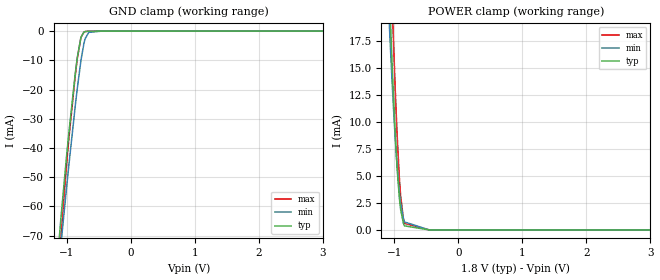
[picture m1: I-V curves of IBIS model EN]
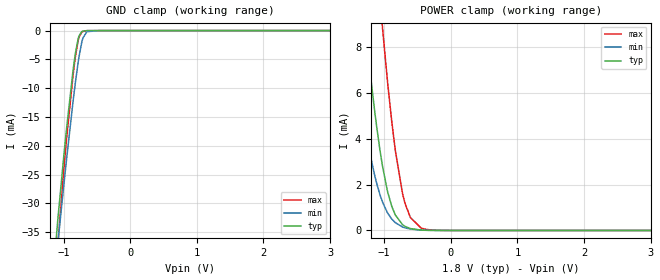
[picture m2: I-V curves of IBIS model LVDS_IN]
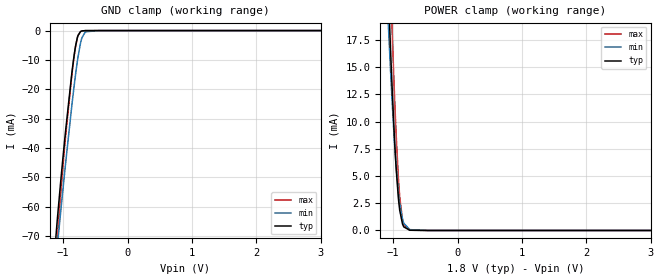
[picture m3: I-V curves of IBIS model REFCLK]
|Texas Instruments Incorporated
| High Performance Single-Synchronous Step-Down Controller
| with Differential Voltage Feedback
| Marketing part#   Digital Voltage Range   Package-type   #pins
| SN65DSI85ZQER   1.65V-1.95   PBGA   64
| SN65DSI85ZQET   1.65V-1.95   PBGA   64
[IBIS Ver]   4.1
[File name]   sn65dsi84.ibs
[File Rev]   1.0
[Date]   1/28/2013
[Source]
| Texas Instruments Incorporated.
| Analog-eLab Design Center, HPA
| 12500 TI Blvd
| Dallas, TX -75243
| e-mail: elab_scm_ibis@list.ti.com
[Notes]   Revision History:
| Rev 1.0: 1/28/2013
| - Initial version of the model
| - Model generated from simulations in TISPICE
| - C_comp although listed in numerical order of value are
|   obtained from varying PVT conditions. For PVT conditions for
|   each specific value refer the buffer description under
|   respective [Model]. IBIS model user is responsible for using
|   appropriate C_comp to simulate for Signal Integrity.
| - Warnings regarding combined Non-monotonicity of various models have been
|   reviewd and considered minor and can be ignored.
| - LVDS outputs have sub models depending on the drive strength/on-chip termination
|   and common mode output level.
|   Please refer to the [Model Selector] section for details.
[Disclaimer]
| This model is designed as an aid for customers of Texas Instruments.
| TI and its licensors and suppliers make no warranties, either expressed
| or implied, with respect to this  model, including the warranties of
| merchantability or fitness for a particular purpose. The model is
| provided solely on an "as is" basis. The entire risk as to its quality
| and performance is with the customer.
[Copyright]
 (C) Copyright 2013 Texas Instruments Incorporated.All rights reserved.
|   SN65DSI84
[Component]   SN65DSI84
[Manufacturer]   TI
[Package]
| variable   typ   min   max
R_pkg   0.1   0.08   0.12
L_pkg   0.7nH   0.56nH   0.84nH
C_pkg   0.1pF   0.08pF   0.12pF
[Pin]  signal_name   model_name   R_pin   L_pin   C_pin
A1   ADDR   ADDR   NA   NA   NA
A2   GND   GND   NA   NA   NA
A3   B_Y0N   LVDS_DATA   NA   NA   NA
A4   B_Y1N   LVDS_DATA   NA   NA   NA
A5   B_Y2N   LVDS_DATA   NA   NA   NA
A6   B_CLKN   LVDS_CLK   NA   NA   NA
A7   B_Y3N   LVDS_DATA   NA   NA   NA
A8   GND   GND   NA   NA   NA
A9   VCC   POWER   NA   NA   NA
B1   EN   EN   NA   NA   NA
B2   RSVD2   NC   NA   NA   NA
B3   B_Y0P   LVDS_DATA   NA   NA   NA
B4   B_Y1P   LVDS_DATA   NA   NA   NA
B5   B_Y2P   LVDS_DATA   NA   NA   NA
B6   B_CLKP   LVDS_CLK   NA   NA   NA
B7   B_Y3P   LVDS_DATA   NA   NA   NA
B8   VCC   POWER   NA   NA   NA
B9   GND   GND   NA   NA   NA
C1   NC   NC   NA   NA   NA
C2   NC   NC   NA   NA   NA
C8   A_Y0P   LVDS_DATA   NA   NA   NA
C9   A_Y0N   LVDS_DATA   NA   NA   NA
D1   NC   NC   NA   NA   NA
D2   NC   NC   NA   NA   NA
D5   GND   GND   NA   NA   NA
D6   VCC   POWER   NA   NA   NA
D8   A_Y1P   LVDS_DATA   NA   NA   NA
D9   A_Y1N   LVDS_DATA   NA   NA   NA
E1   NC   NC   NA   NA   NA
E2   NC   NC   NA   NA   NA
E4   GND   GND   NA   NA   NA
E5   VCC   POWER   NA   NA   NA
E6   VCC   POWER   NA   NA   NA
E8   A_Y2P   LVDS_DATA   NA   NA   NA
E9   A_Y2N   LVDS_DATA   NA   NA   NA
F1   NC   NC   NA   NA   NA
F2   NC   NC   NA   NA   NA
F4   GND   GND   NA   NA   NA
F5   GND   GND   NA   NA   NA
F6   VCC   POWER   NA   NA   NA
F8   A_CLKP   LVDS_CLK   NA   NA   NA
F9   A_CLKN   LVDS_CLK   NA   NA   NA
G1   NC   NC   NA   NA   NA
G2   NC   NC   NA   NA   NA
G8   A_Y3P   LVDS_DATA   NA   NA   NA
G9   A_Y3N   LVDS_DATA   NA   NA   NA
H1   SCL   SCL   NA   NA   NA
H2   REFCLK   REFCLK   NA   NA   NA
H3   DAP0P   LVDS_IN   NA   NA   NA
H4   DAP1P   LVDS_IN   NA   NA   NA
H5   DACP   LVDS_IN   NA   NA   NA
H6   DA2P   LVDS_IN   NA   NA   NA
H7   DAP3P   LVDS_IN   NA   NA   NA
H8   RSVD1   NC   NA   NA   NA
H9   GND   GND   NA   NA   NA
J1   SDA   SDA   NA   NA   NA
J2   VCC   POWER   NA   NA   NA
J3   DA0N   LVDS_IN   NA   NA   NA
J4   DA1N   LVDS_IN   NA   NA   NA
J5   DACN   LVDS_IN   NA   NA   NA
J6   DA2N   LVDS_IN   NA   NA   NA
J7   DA3N   LVDS_IN   NA   NA   NA
J8   VCORE   POWER   NA   NA   NA
J9   IRQ   IRQ   NA   NA   NA
[Diff Pin]  inv_pin  vdiff  tdelay_typ tdelay_min tdelay_max
H3   J3   100mV   NA   NA   NA
H4   J4   100mV   NA   NA   NA
H6   J6   100mV   NA   NA   NA
H7   J7   100mV   NA   NA   NA
H5   J5   100mV   NA   NA   NA
C8   C9   NA   NA   NA   NA
D8   D9   NA   NA   NA   NA
E8   E9   NA   NA   NA   NA
G8   G9   NA   NA   NA   NA
F8   F9   NA   NA   NA   NA
B3   A3   NA   NA   NA   NA
B4   A4   NA   NA   NA   NA
B5   A5   NA   NA   NA   NA
B7   A7   NA   NA   NA   NA
B6   A6   NA   NA   NA   NA
|   Model Selectors
[Model Selector]  LVDS_DATA
lvds_1p2_term100_11 lvds w/ 100ohm diff term and high strength and 1.2v Vcm
lvds_1p2_term100_00 lvds w/ 100ohm diff term and low strength and 1.2v Vcm
lvds_0p9_term100_11 lvds w/ 100ohm diff term and high strength and 0.9v Vcm
lvds_0p9_term100_00 lvds w/ 100ohm diff term and low strength and 0.9v Vcm
lvds_1p2_term200_11 lvds w/ 200ohm diff term and high strength and 1.2v Vcm
lvds_1p2_term200_00 lvds w/ 200ohm diff term and low strength and 1.2v Vcm
lvds_0p9_term200_11 lvds w/ 200ohm diff term and high strength and 0.9v Vcm
lvds_0p9_term200_00 lvds w/ 200ohm diff term and low strength and 0.9v Vcm
LVDS_PD   lvds driver in tri-state with 1k pull down
[Model Selector]  LVDS_CLK
lvds_clk_1p2_term100_11 clk drv w/ 100ohm diff term w/ high strength and 1.2v Vcm
lvds_clk_1p2_term100_00 clk drv w/ 100ohm diff term w/ low strength and 1.2v Vcm
lvds_clk_0p9_term100_11 clk drv w/ 100ohm diff term w/ high strength and 0.9v Vcm
lvds_clk_0p9_term100_00 clk drv w/ 100ohm diff term w/ low strength and 0.9v Vcm
lvds_clk_1p2_term200_11 clk drv w/ 200ohm diff term w/ high strength and 1.2v Vcm
lvds_clk_1p2_term200_00 clk drv w/ 200ohm diff term w/ low strength and 1.2v Vcm
lvds_clk_0p9_term200_11 clk drv w/ 200ohm diff term w/ high strength and 0.9v Vcm
lvds_clk_0p9_term200_00 clk drv w/ 200ohm diff term w/ low strength and 0.9v Vcm
LVDS_PD   clk driver in tri-state with 1k pull down
| Models and submodels in the file (24): ADDR (I/O), EN (Input), IRQ (Output), LVDS_IN (Input), LVDS_PD (Terminator), REFCLK (Input), SCL (Input), SDA (I/O_open_drain), lvds_0p9_term100_00 (Output), lvds_0p9_term100_11 (Output), lvds_0p9_term200_00 (Output), lvds_0p9_term200_11 (Output), lvds_1p2_term100_00 (Output), lvds_1p2_term100_11 (Output), lvds_1p2_term200_00 (Output), lvds_1p2_term200_11 (Output), lvds_clk_0p9_term100_00 (Output), lvds_clk_0p9_term100_11 (Output), lvds_clk_0p9_term200_00 (Output), lvds_clk_0p9_term200_11 (Output), lvds_clk_1p2_term100_00 (Output), lvds_clk_1p2_term100_11 (Output), lvds_clk_1p2_term200_00 (Output), lvds_clk_1p2_term200_11 (Output)
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|   Model
[Model]   EN
Model_type   Input
Vinl = 0.54
Vinh = 1.26
|   typ   min   max
C_comp   0.1884pF   0.1127pF   0.2695pF
[Voltage Range]   1.8   1.65   1.95
[Temperature Range]   27   125   -40
[Power Clamp Reference]   1.8   1.65   1.95
[GND Clamp Reference]   -0   -0   -0
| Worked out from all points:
|   GND clamp passes 1 mA (typ) near -0.75 V on its own axis
|   POWER clamp passes 1 mA (typ) near -0.87 V on its own axis
[GND Clamp]
|   Voltage   I(typ)   I(min)   I(max)
-1.8V     -308mA     -292.1mA   -326.9mA
-1.141V   -77.88mA   -84.93mA   -86.8mA
-1.093V   -64.81mA   -73.77mA   -71.46mA
-1.006V   -43.97mA   -54.68mA   -47mA
-963mV    -34.36mA   -45.43mA   -36.29mA
-849.6mV  -11.75mA   -22.57mA   -12.28mA
-833.4mV  -9.068mA   -19.57mA   -9.452mA
-779.4mV  -2.443mA   -10.49mA   -2.453mA
-725.4mV  -293.5uA   -3.805mA   -304.2uA
-655.2mV  -23.86uA   -437.3uA   -34.42uA
-450mV    -11.25uA   -8.997uA   -14.64uA
3.595V    0A         0A         0A
[POWER Clamp]
|   Voltage   I(typ)   I(min)   I(max)
-1.8V     160.5mA    134.1mA    187.1mA
-1.071V   21.35mA    18.46mA    28.35mA
-1.066V   20.5mA     17.78mA    27.33mA
-1.033V   15.58mA    13.84mA    21.41mA
-1.012V   12.54mA    11.41mA    17.66mA
-963mV    6.678mA    6.677mA    10.12mA
-919.8mV  3.037mA    3.574mA    4.952mA
-898.2mV  1.865mA    2.464mA    3.117mA
-855mV    602.7uA    1.05mA     994.1uA
-838.8mV  381.2uA    741.1uA    611.7uA
-450mV    2.251uA    1.957uA    2.744uA
3.595V    0A         0A         0A
|   Model
[Model]   LVDS_IN
Model_type   Input
Vinl = 0.55
Vinh = 0.88
|   typ   min   max
C_comp   0.2021pF   0.1391pF   0.2894pF
[Voltage Range]   1.8   1.65   1.95
[Temperature Range]   27   125   -40
[Power Clamp Reference]   1.8   1.65   1.95
[GND Clamp Reference]   -0   -0   -0
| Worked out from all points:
|   GND clamp passes 1 mA (typ) near -0.77 V on its own axis
|   POWER clamp passes 1 mA (typ) near -0.88 V on its own axis
[GND Clamp]
|   Voltage   I(typ)   I(min)   I(max)
-1.8V     -157.2mA   -148.1mA   -169.7mA
-1.136V   -39.5mA    -42.69mA   -45.17mA
-1.087V   -32.88mA   -37.02mA   -37.3mA
-995.4mV  -21.59mA   -26.69mA   -23.97mA
-952.2mV  -16.67mA   -22mA      -18.44mA
-860.4mV  -7.155mA   -12.54mA   -8.035mA
-822.6mV  -3.925mA   -8.98mA    -4.498mA
-779.4mV  -1.325mA   -5.345mA   -1.604mA
-725.4mV  -167.9uA   -1.945mA   -265.1uA
-649.8mV  -6.948uA   -183.8uA   -17.24uA
-450mV    -177.8nA   -227.6nA   -350.8nA
3.595V    0A         0A         0A
[POWER Clamp]
|   Voltage   I(typ)   I(min)   I(max)
-1.8V     26.26mA    16.82mA    40.22mA
-1.519V   16.37mA    9.509mA    28.04mA
-1.427V   13.34mA    7.397mA    24.18mA
-1.282V   8.867mA    4.489mA    18.25mA
-1.147V   5.295mA    2.45mA     13.08mA
-1.022V   2.757mA    1.221mA    8.741mA
-887.4mV  1.06mA     500.7uA    4.771mA
-833.4mV  676.8uA    340.7uA    3.496mA
-725.4mV  256.1uA    152.8uA    1.621mA
-606.6mV  82.84uA    61.3uA     563.7uA
-331.2mV  6.105uA    7.007uA    33.99uA
3.595V    0A         0A         0A
|   Model
[Model]   REFCLK
Model_type   Input
Vinl = 0.54
Vinh = 1.26
|   typ   min   max
C_comp   0.188pF   0.113pF   0.270pF
[Voltage Range]   1.8   1.65   1.95
[Temperature Range]   27   125   -40
[Power Clamp Reference]   1.8   1.65   1.95
[GND Clamp Reference]   -0   -0   -0
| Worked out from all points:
|   GND clamp passes 1 mA (typ) near -0.75 V on its own axis
|   POWER clamp passes 1 mA (typ) near -0.87 V on its own axis
[GND Clamp]
|   Voltage   I(typ)   I(min)   I(max)
-1.8V     -308mA     -292.1mA   -326.9mA
-1.141V   -77.87mA   -84.93mA   -86.79mA
-1.087V   -63.42mA   -72.55mA   -69.8mA
-1.033V   -50.21mA   -60.55mA   -54.19mA
-963mV    -34.35mA   -45.43mA   -36.28mA
-860.4mV  -13.64mA   -24.61mA   -14.26mA
-817.2mV  -6.639mA   -16.67mA   -6.881mA
-779.4mV  -2.431mA   -10.48mA   -2.438mA
-725.4mV  -281.1uA   -3.796mA   -288.1uA
-655.2mV  -11.59uA   -427.7uA   -18.55uA
-450mV    -450.2pA   -165.7nA   -4.233nA
3.595V    0A         0A         0A
[POWER Clamp]
|   Voltage   I(typ)   I(min)   I(max)
-1.8V     160.5mA    134.1mA    187.1mA
-1.071V   21.35mA    18.46mA    28.34mA
-1.044V   17.18mA    15.11mA    23.34mA
-1.033V   15.58mA    13.84mA    21.4mA
-1.012V   12.54mA    11.4mA     17.66mA
-963mV    6.674mA    6.673mA    10.11mA
-919.8mV  3.033mA    3.571mA    4.947mA
-898.2mV  1.861mA    2.46mA     3.112mA
-833.4mV  322.4uA    654.5uA    513uA
-741.6mV  20.48uA    76.69uA    25.35uA
-450mV    1.114nA    64.12nA    495.4pA
3.595V    0A         0A         0A
